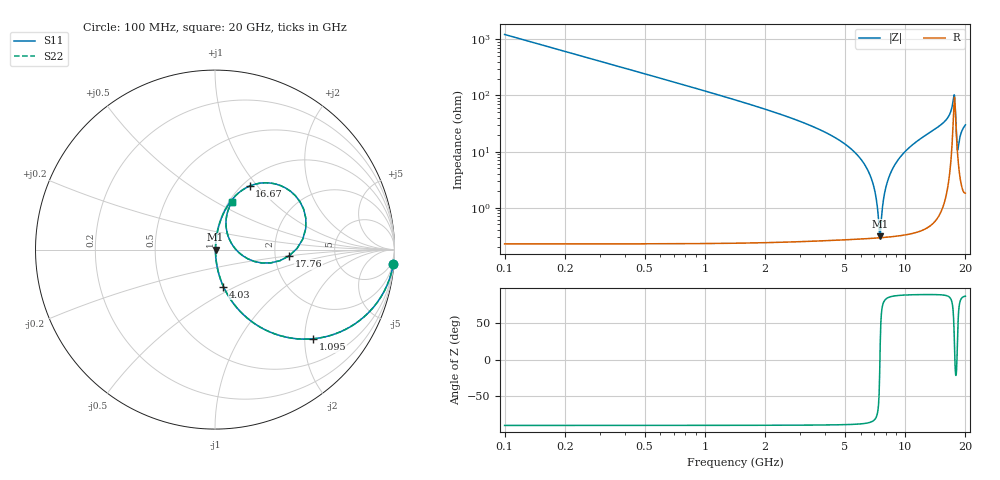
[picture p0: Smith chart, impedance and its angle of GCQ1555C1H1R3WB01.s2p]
!Murata Part Number: GCQ1555C1H1R3WB01
!These Parameters are Measured in Series Mode Connection
!Data Generated on Jan 08, 2026
!  o--ll--o
!Port1  Port2
!  o------o
!Operation Temp=25[degC], DC Bias Voltage=0[V]
!Freq. Start=100[MHz] Stop=20[GHz] 401[Steps]
# Hz S RI R 50
!Freq.(Hz) S11(Real) S11(Imag) S21(Real) S21(Imag) S12(Real) S12(Imag) S22(Real) S22(Imag)
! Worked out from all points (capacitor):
!   401 points, 100 MHz to 20 GHz, reference 50 ohm
!   read as one part in series: C = 1.3 pF near 199.5 MHz
!   lowest |Z| = 307 mohm at 7.463 GHz (marker M1)
!   series resonance near 7.486 GHz, so ESL is about 350 pH
!   S11 on the Smith chart (normalised r, x): 100 MHz: 1, -24; 1.095 GHz: 1.00, -2.19; 4.03 GHz: 1.01, -0.43; 16.67 GHz: 1.08, +0.91; 17.76 GHz: 2.40, -0.20; 20 GHz: 1.04, +0.60
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1e8  0.9934 -0.0812  0.00664 0.0812  0.00664 0.0812  0.9934 -0.0812
4.4825e8  0.8808 -0.3236  0.1192 0.3236  0.1192 0.3236  0.8808 -0.3236
1.095e9  0.5449 -0.4969  0.4551 0.4969  0.4551 0.4969  0.5449 -0.4969
2.04025e9  0.2371 -0.4232  0.7629 0.4232  0.7629 0.4232  0.2371 -0.4232
3.43325e9  0.0759 -0.2604  0.9241 0.2604  0.9241 0.2604  0.0759 -0.2604
4.03025e9  0.0471 -0.2059  0.9529 0.2059  0.9529 0.2059  0.0471 -0.2059
5.7715e9  0.0102 -0.0858  0.9898 0.0858  0.9898 0.0858  0.0102 -0.0858
6.7665e9  0.00393 -0.0334  0.9961 0.0334  0.9961 0.0334  0.00393 -0.0334
7.1645e9  0.00307 -0.0145  0.9969 0.0145  0.9969 0.0145  0.00307 -0.0145
7.463e9  0.00289 -0.00102  0.9971 0.00102  0.9971 0.00102  0.00289 -0.00102
7.5625e9  0.00291 0.00337  0.9971 -0.00337  0.9971 -0.00337  0.00291 0.00337
7.861e9  0.00319 0.0162  0.9968 -0.0162  0.9968 -0.0162  0.00319 0.0162
8.259e9  0.00405 0.0327  0.9959 -0.0327  0.9959 -0.0327  0.00405 0.0327
1.005e10  0.0134 0.1  0.9866 -0.1  0.9866 -0.1  0.0134 0.1
1.338325e10  0.0513 0.2103  0.9487 -0.2103  0.9487 -0.2103  0.0513 0.2103
1.666675e10  0.1923 0.3535  0.8077 -0.3535  0.8077 -0.3535  0.1923 0.3535
1.67165e10  0.2002 0.3567  0.7998 -0.3567  0.7998 -0.3567  0.2002 0.3567
1.73135e10  0.3932 0.3433  0.6068 -0.3433  0.6068 -0.3433  0.3932 0.3433
1.776125e10  0.4131 -0.0348  0.5869 0.0348  0.5869 0.0348  0.4131 -0.0348
1.825875e10  0.0892 0.0389  0.9108 -0.0389  0.9108 -0.0389  0.0892 0.0389
1.9005e10  0.0652 0.1898  0.9348 -0.1898  0.9348 -0.1898  0.0652 0.1898
2e10  0.0954 0.265  0.9046 -0.265  0.9046 -0.265  0.0954 0.265
